FUNCTION "COM_GEN" : VOID
TITLE =GENERAL MANAGEMENT
AUTHOR : DM
VERSION : 0.1

BEGIN
NETWORK
TITLE =INSERT COMMAND
//AUXILIARY ON
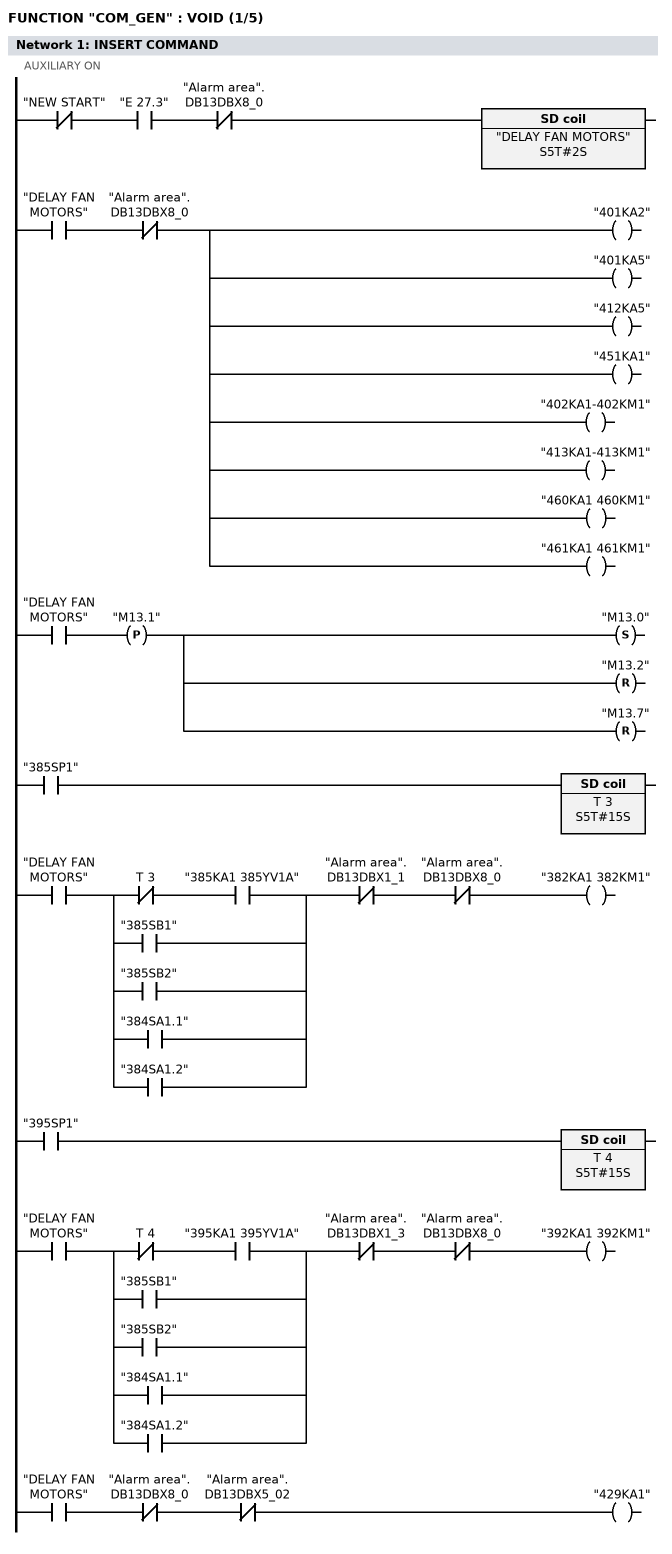
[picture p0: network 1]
      UN    "NEW START";
      U     "E      27.3";
      UN    "Alarm area".DB13DBX8_0;
      L     S5T#2S;
      SE    "DELAY FAN MOTORS";

      U     "DELAY FAN MOTORS";
      UN    "Alarm area".DB13DBX8_0;
      =     "401KA2";
      =     "401KA5";
      =     "412KA5";
      =     "451KA1";
      =     "402KA1-402KM1";
      =     "413KA1-413KM1";
      =     "460KA1 460KM1";
      =     "461KA1 461KM1";

      U     "DELAY FAN MOTORS";
      FP    "M13.1";
      S     "M13.0";
      R     "M13.2";
      R     "M13.7";

//      UN    "ALARMS DATA".DB13DBX4_02
      U     "385SP1";
      L     S5T#15S;
      SE    T      3;

      U     "DELAY FAN MOTORS";
      U(    ;
      UN    T      3;
      U     "385KA1 385YV1A";
      O     "385SB1";
      O     "385SB2";
      O     "384SA1.1";
      O     "384SA1.2";
      )     ;
      UN    "Alarm area".DB13DBX1_1;
      UN    "Alarm area".DB13DBX8_0;
      =     "382KA1 382KM1";

//      UN    "ALARMS DATA".DB13DBX4_04
      U     "395SP1";
      L     S5T#15S;
      SE    T      4;


      U     "DELAY FAN MOTORS";
      U(    ;
      UN    T      4;
      U     "395KA1 395YV1A";
      O     "385SB1";
      O     "385SB2";
      O     "384SA1.1";
      O     "384SA1.2";
      )     ;
      UN    "Alarm area".DB13DBX1_3;
      UN    "Alarm area".DB13DBX8_0;
      =     "392KA1 392KM1";

      U     "DELAY FAN MOTORS";
      UN    "Alarm area".DB13DBX8_0;
      UN    "Alarm area".DB13DBX5_02;
      =     "429KA1";

NETWORK
TITLE =ENABLE TD17
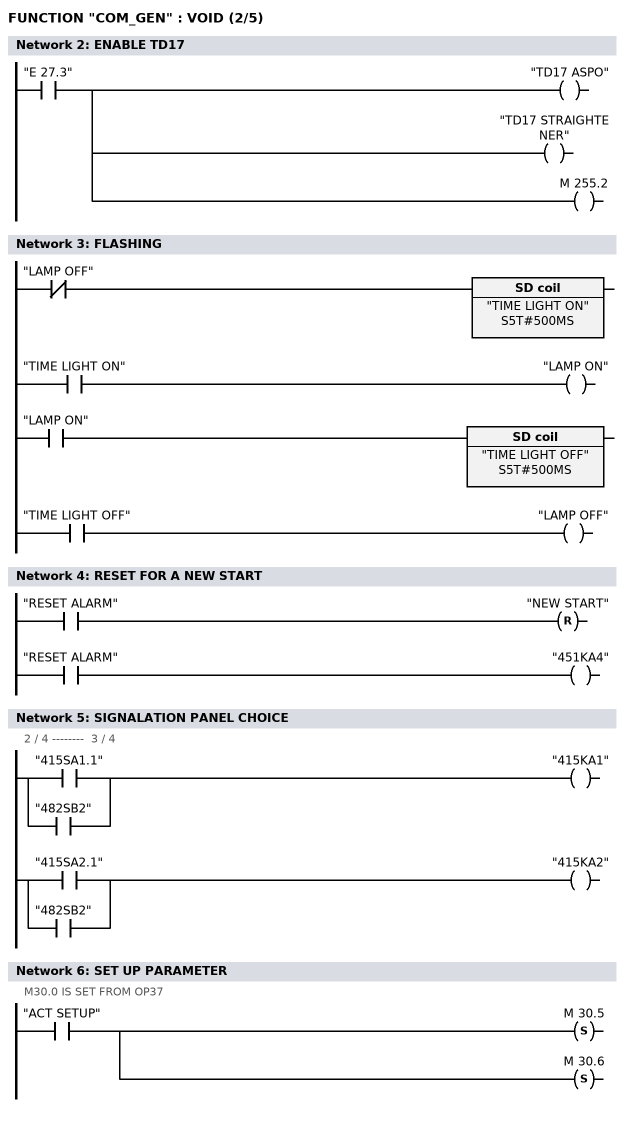
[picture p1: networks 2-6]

      U     "E      27.3";
      =     "TD17 ASPO";
      =     "TD17 STRAIGHTENER";
      =     M    255.2;
NETWORK
TITLE =FLASHING

      UN    "LAMP OFF";
      L     S5T#500MS;
      SE    "TIME LIGHT ON";
      NOP   0;
      NOP   0;
      NOP   0;
      U     "TIME LIGHT ON";
      =     "LAMP ON";

      U     "LAMP ON";
      L     S5T#500MS;
      SE    "TIME LIGHT OFF";
      NOP   0;
      NOP   0;
      NOP   0;
      U     "TIME LIGHT OFF";
      =     "LAMP OFF";


NETWORK
TITLE =RESET FOR A NEW START

// ENABLE AUXILIARY
      U     "RESET ALARM";
      R     "NEW START";

// RESET OF ABB MOTOR FAILURE
      U     "RESET ALARM";
      =     "451KA4";

NETWORK
TITLE =SIGNALATION PANEL CHOICE
//2 / 4 --------  3 / 4

      U     "415SA1.1";
      O     ;
      U     "482SB2";
      =     "415KA1";

      U     "415SA2.1";
      O     ;
      U     "482SB2";
      =     "415KA2";

NETWORK
TITLE =SET UP PARAMETER
//M30.0 IS SET FROM OP37
      U     "ACT SETUP";
      S     M     30.5;
      S     M     30.6;
NETWORK
TITLE =SET UP PARAMETER
//RESET M30.0 WHEN ALL IN POSITION
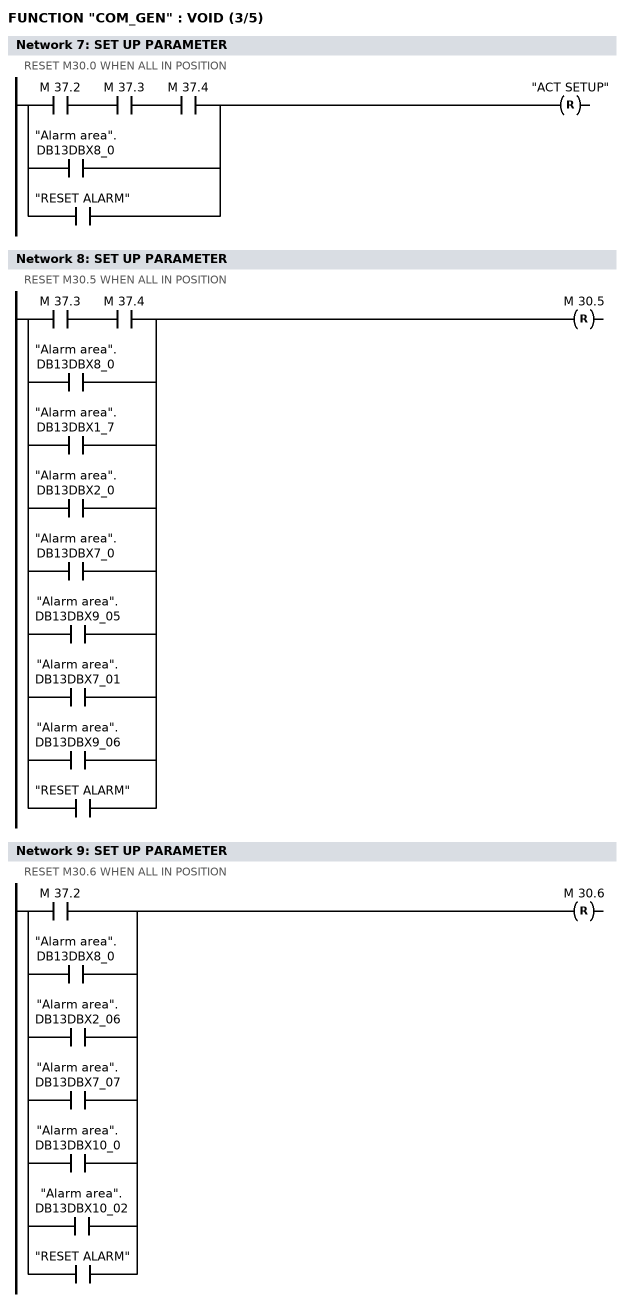
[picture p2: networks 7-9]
      U     M     37.2;
      U     M     37.3;
      U     M     37.4;
      O     "Alarm area".DB13DBX8_0;
      O     "RESET ALARM";
      R     "ACT SETUP";

NETWORK
TITLE =SET UP PARAMETER
//RESET M30.5 WHEN ALL IN POSITION
      U     M     37.3;
      U     M     37.4;
      O     "Alarm area".DB13DBX8_0;
      O     "Alarm area".DB13DBX1_7;
      O     "Alarm area".DB13DBX2_0;
      O     "Alarm area".DB13DBX7_0;
      O     "Alarm area".DB13DBX9_05;
      O     "Alarm area".DB13DBX7_01;
      O     "Alarm area".DB13DBX9_06;
      O     "RESET ALARM";
      R     M     30.5;

NETWORK
TITLE =SET UP PARAMETER
//RESET M30.6 WHEN ALL IN POSITION
      U     M     37.2;
      O     "Alarm area".DB13DBX8_0;
      O     "Alarm area".DB13DBX2_06;
      O     "Alarm area".DB13DBX7_07;
      O     "Alarm area".DB13DBX10_0;
      O     "Alarm area".DB13DBX10_02;
      O     "RESET ALARM";
      R     M     30.6;

NETWORK
TITLE =ALARM
//321SB2
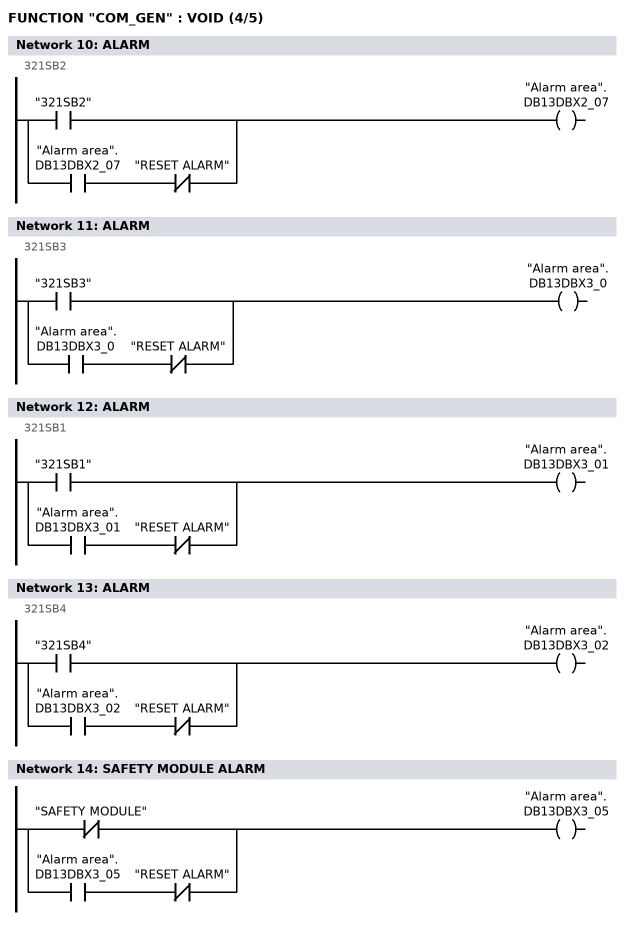
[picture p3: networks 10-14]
      O     "321SB2";
      O     ;
      U     "Alarm area".DB13DBX2_07;
      UN    "RESET ALARM";
      =     "Alarm area".DB13DBX2_07;

NETWORK
TITLE =ALARM
// 321SB3
      O     "321SB3";
      O     ;
      U     "Alarm area".DB13DBX3_0;
      UN    "RESET ALARM";
      =     "Alarm area".DB13DBX3_0;

NETWORK
TITLE =ALARM
//321SB1
      O     "321SB1";
      O     ;
      U     "Alarm area".DB13DBX3_01;
      UN    "RESET ALARM";
      =     "Alarm area".DB13DBX3_01;

NETWORK
TITLE =ALARM
//321SB4
      O     "321SB4";
      O     ;
      U     "Alarm area".DB13DBX3_02;
      UN    "RESET ALARM";
      =     "Alarm area".DB13DBX3_02;

NETWORK
TITLE =SAFETY MODULE ALARM

      ON    "SAFETY MODULE";
      O     ;
      U     "Alarm area".DB13DBX3_05;
      UN    "RESET ALARM";
      =     "Alarm area".DB13DBX3_05;

NETWORK
TITLE =EMERGENCY ALARM
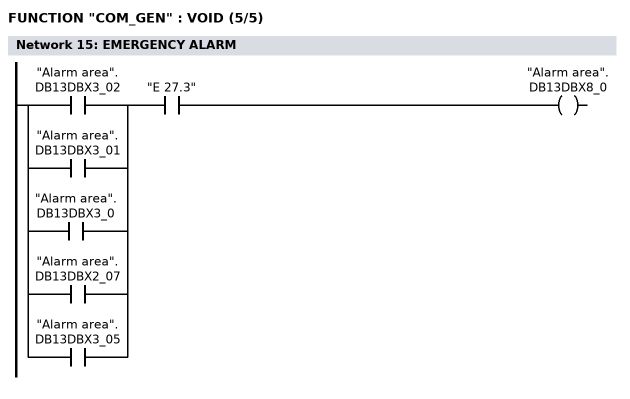
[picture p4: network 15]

      U(    ;
      O     "Alarm area".DB13DBX3_02;
      O     "Alarm area".DB13DBX3_01;
      O     "Alarm area".DB13DBX3_0;
      O     "Alarm area".DB13DBX2_07;
      O     "Alarm area".DB13DBX3_05;
      )     ;
      U     "E      27.3";
      =     "Alarm area".DB13DBX8_0;
END_FUNCTION

